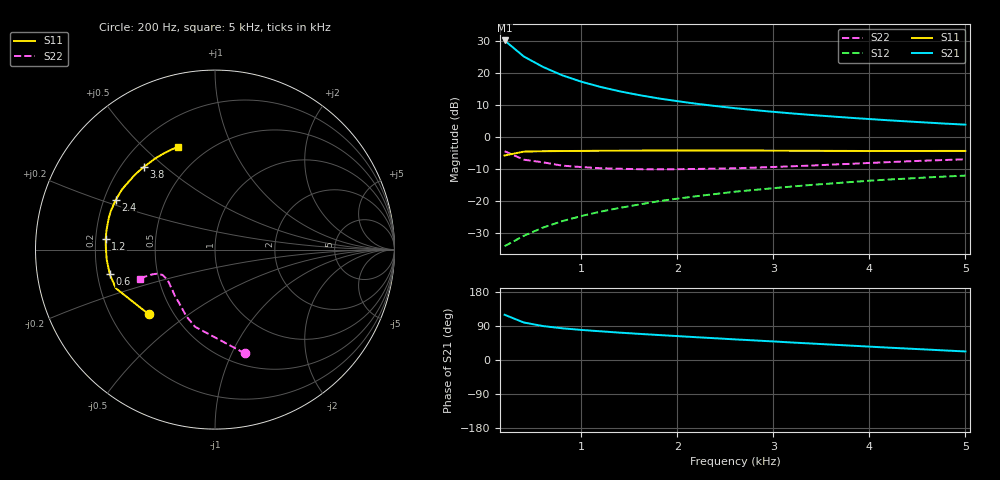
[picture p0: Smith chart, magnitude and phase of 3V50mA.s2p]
#  HZ  S  MA  R  50.0000
! Device:MCH4020
! Bias:VCE=3V, IC=50mA
!MHZ	S11(MAG/ANG)		S21(MAG/ANG)		S12(MAG/ANG)		S22(MAG/ANG)
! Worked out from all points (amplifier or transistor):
!   25 points, 200 Hz to 5 kHz, reference 50 ohm
!   highest |S21| = 30.1 dB at 200 Hz (marker M1)
!   |S21| within 3 dB of that: start of sweep to 320.1 Hz
!   unconditionally stable (mu >= 1): 2.364 kHz to 2.504 kHz; 2.645 kHz to 3.389 kHz
!   at 1 kHz: K = 0.89, MSG = 20.9 dB, |S12| = -24.6 dB
!   at 2.6 kHz: K = 1.00, MSG = 13.0 dB, |S12| = -17.0 dB
!   at 5 kHz: K = 0.96, MSG = 7.9 dB, |S12| = -12.0 dB
!   S11 on the Smith chart (normalised r, x): 200 Hz: 0.37, -0.36; 600 Hz: 0.25, -0.11; 1.2 kHz: 0.24, +0.05; 2.4 kHz: 0.25, +0.22; 3.8 kHz: 0.29, +0.43; 5 kHz: 0.35, +0.64
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200  0.516 -135.8  31.91 119.4  0.02 59.2  0.602 -73.9
400  0.593 -158.7  17.95 99.0  0.029 60.4  0.444 -104.5
600  0.602 -166.8  12.35 89.5  0.039 63.6  0.404 -113.3
800  0.606 -174.8  9.16 83.7  0.049 65.9  0.359 -123.7
1000  0.608 179.2  7.261 79.3  0.059 67.0  0.341 -131.0
1200  0.612 174.4  6.025 75.7  0.069 67.5  0.327 -136.6
1400  0.614 170.2  5.149 72.2  0.079 67.4  0.321 -140.6
1600  0.615 166.4  4.503 69.0  0.089 67.2  0.316 -144.0
1800  0.618 162.9  4.004 66.0  0.1 66.4  0.314 -146.9
2000  0.619 159.8  3.619 63.1  0.11 65.8  0.316 -149.3
2200  0.618 156.5  3.299 60.1  0.12 64.9  0.319 -151.3
2400  0.618 153.5  3.035 57.3  0.13 63.9  0.322 -152.9
2600  0.617 150.5  2.816 54.4  0.141 62.7  0.326 -154.5
2800  0.617 147.4  2.63 51.7  0.15 61.6  0.334 -155.5
3000  0.614 144.2  2.469 49.0  0.16 60.3  0.342 -156.7
3200  0.611 141.0  2.328 46.1  0.17 58.9  0.351 -157.4
3400  0.611 137.6  2.204 43.4  0.18 57.5  0.36 -157.9
3800  0.608 130.8  1.995 38.0  0.199 54.7  0.383 -158.6
4200  0.607 123.6  1.824 32.6  0.218 51.5  0.407 -158.8
4400  0.607 120.1  1.749 30.1  0.226 49.9  0.419 -158.9
4800  0.608 113.0  1.616 25.0  0.243 46.8  0.44 -158.9
5000  0.608 109.6  1.56 22.6  0.251 45.2  0.45 -159.0
